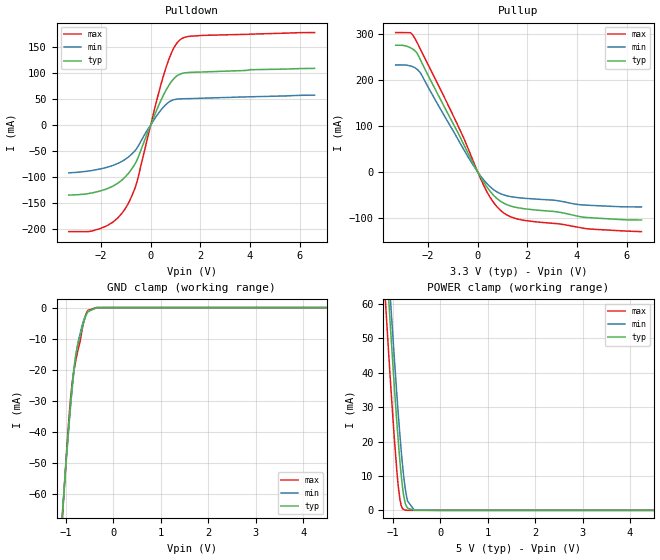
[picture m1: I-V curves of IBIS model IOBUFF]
[IBIS Ver]  4.2
[File Name] trad-nodal-pinmapping.ibs
[File Rev]  1.0
[Date]   01/21/2008
[Source]   This information is for demonstration purposes only.
[Notes]   The following information corresponds to no actual device.
[Disclaimer]   No license, express or implied, by estoppel or
  otherwise, to any intellectual property rights is granted
  by this document.
[Copyright]   Copyright (C) 2008, GEIA and the IBIS Open Forum
[Component]   Traditional_Nodal_Pinmapping
[Manufacturer]  IBIS Open Forum
[Package]   | this section is overridden by [Package Model]
|   typ   min   max
R_pkg   0.00mOhm   0.00mOhm   0.00mOhm
L_pkg   0.0nH   0.00nH   0.00nH
C_pkg   0.0pF   0.00pF   0.00pF
[Pin]   signal_name model_name R_pin  L_pin  C_pin
| R_, L_ and C_pin are also overridden by [Package Model]
A1   IOPIN2   IOBUFF   2m   4n   1p
A4   VCC   POWER   2m   4n   1p
A5   VSS   GND   2m   4n   1p
| To make this work under ICM with [Pin Mapping], you would connect
| a node map or a pin map using the names A1, A4 and A5 at the pin end,
| with A1 and the rail names power_rail and gnd_rail at the die end, if the
| supply for the buffer comes from the two supply pins named.
[Package Model]   trad-nodal-pinmapping.icm
| ICM usage with IBIS package models requires the use of a [Package Model]
| with an .icm extension
[Pin Mapping] pulldown_ref pullup_ref gnd_clamp_ref   power_clamp_ref
A1   gnd_rail   power_rail  gnd_rail   power_rail
A4   NC   power_rail  NC   NC
A5   gnd_rail   NC   NC   NC
| Models and submodels in the file (1): IOBUFF (I/O)
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[Model]   IOBUFF
Model_type   I/O
Vinl = 0.99V
Vinh = 1.650V
Vref = 0.000V
Cref = 10.000pF
Rref = 25.000Ohm
Vmeas = 1.0
|   typ   min   max
C_comp   2.115pF   1.917pF   2.360pF
[Voltage Range]   3.300V   3.135V   3.465V
[Power Clamp Reference]   5.000V   4.750V   5.250V
[Temperature Range]   60.0   110.0   -10.0
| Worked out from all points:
|   slope of the pulldown table from 0 to 0.495 V, typ, clamps not added: 8.87 ohm
|   slope of the pullup table from 0 to 0.495 V, typ, clamps not added: 11.8 ohm
|   GND clamp passes 1 mA (typ) near -0.50 V on its own axis
|   POWER clamp passes 1 mA (typ) near -0.71 V on its own axis
[Pulldown]
|   Voltage   I(typ)   I(min)   I(max)
-3.3V     -134.6mA   -91.87mA   -204.8mA
-2.48V    -131.4mA   -88.14mA   -204.6mA
-1.78V    -122.8mA   -81.39mA   -193.8mA
-1.34V    -112.1mA   -74.04mA   -179mA
-985mV    -97.54mA   -64.49mA   -157.5mA
-555mV    -67.45mA   -44.34mA   -109mA
200mV     24.21mA    15.11mA    39.53mA
615mV     66.89mA    39.5mA     110.4mA
915mV     88.29mA    48.43mA    146.6mA
1.22V     98.53mA    50.37mA    165.2mA
2.135V    102.1mA    51.68mA    172.3mA
6.6V      108.9mA    57.44mA    177.7mA
[GND Clamp]
|   Voltage   I(typ)   I(min)   I(max)
-4.995V   -813.8mA   -713.5mA   -1A
-1.075V   -66.47mA   -65.64mA   -67.69mA
-1.06V    -63.08mA   -62.47mA   -63.84mA
-965mV    -42.57mA   -43.21mA   -41.14mA
-900mV    -30.04mA   -31.2mA    -28.54mA
-845mV    -21.21mA   -22.32mA   -21.43mA
-795mV    -15.36mA   -15.8mA    -17.09mA
-740mV    -11.29mA   -10.72mA   -13.2mA
-665mV    -6.864mA   -5.986mA   -7.473mA
-575mV    -2.403mA   -2.21mA    -1.982mA
-355mV    -10.71uA   -19.19uA   -2.442uA
9.995V    0A         0A         0A
[Pullup]
|   Voltage   I(typ)   I(min)   I(max)
-3.3V     276.5mA    233.4mA    304.1mA
-2.705V   270.9mA    231.2mA    303.8mA
-2.56V    265.9mA    228.3mA    294.3mA
-2.315V   245.8mA    216.9mA    268.8mA
-775mV    83.6mA     69.25mA    98.88mA
0V        109nA      136.8nA    52.28nA
510mV     -43.04mA   -33mA      -56.32mA
985mV     -66.51mA   -49.18mA   -87.1mA
1.4V      -75.83mA   -54.83mA   -99.76mA
1.95V     -81.2mA    -58.11mA   -106.7mA
4.285V    -99.27mA   -72.57mA   -123.5mA
6.6V      -105.3mA   -76.73mA   -130.7mA
[POWER Clamp]
|   Voltage   I(typ)   I(min)   I(max)
-4.995V   780mA      749.5mA    799.7mA
-1.155V   76.37mA    84.27mA    60.39mA
-1.125V   69.55mA    77.55mA    53.61mA
-1.06V    55.11mA    63.28mA    39.37mA
-1.04V    50.78mA    58.98mA    35.12mA
-965mV    35.11mA    43.34mA    20.06mA
-880mV    18.99mA    26.9mA     6.208mA
-825mV    10.28mA    17.46mA    1.438mA
-745mV    2.374mA    6.872mA    78.88uA
-690mV    625.5uA    2.682mA    19.99uA
-550mV    23.83uA    120.7uA    1.561uA
9.995V    0A         0A         0A
[Ramp]
R_load = 60.00Ohm
|   typ   min   max
dV/dt_r   1.649V/481.483ps   1.467V/1.077ns  1.812V/299.994ps
dV/dt_f   1.730V/957.432ps   1.487V/2.240ns  1.915V/549.942ps
